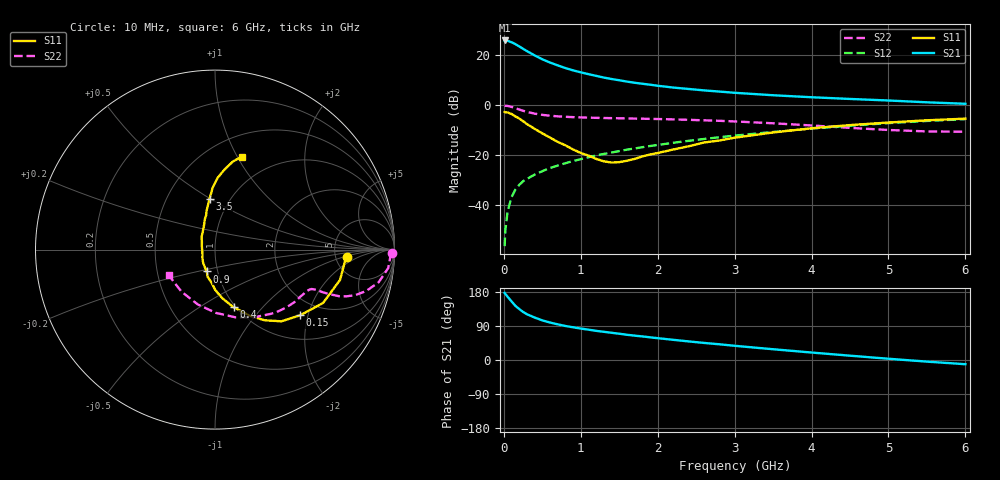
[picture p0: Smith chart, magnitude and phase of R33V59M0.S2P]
! SIEMENS Small Signal Semiconductors
! BFR181
! Si NPN RF Bipolar Junction Transistor in SOT23
! VCE = 3.5 V  IC = 9 mA
! Common Emitter S-Parameters:  May  1996
# GHz  S  MA  R  50
!  f  S11  S21  S12  S22
! GHz  MAG  ANG  MAG  ANG  MAG  ANG  MAG  ANG
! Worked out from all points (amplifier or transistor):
!   36 points, 10 MHz to 6 GHz, reference 50 ohm
!   highest |S21| = 26.0 dB at 10 MHz (marker M1)
!   |S21| within 3 dB of that: start of sweep to 232.2 MHz
!   unconditionally stable (mu >= 1): 819.5 MHz to 2.688 GHz
!   at 250 MHz: K = 0.58, MSG = 26.5 dB, |S12| = -30.4 dB
!   at 1.4 GHz: K = 1.06, MAG = 13.2 dB, |S12| = -18.9 dB
!   at 6 GHz: K = 0.85, MSG = 3.1 dB, |S12| = -5.5 dB
!   S11 on the Smith chart (normalised r, x): 10 MHz: 6.36, -1.06; 150 MHz: 1.56, -1.79; 400 MHz: 0.98, -0.71; 900 MHz: 0.89, -0.22; 3.5 GHz: 0.80, +0.50; 6 GHz: 0.72, +1.05
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0.01  0.735 -3.0  19.95 177.0  0.0015 82.7  0.9858 -1.1
0.02  0.7261 -5.6  19.92 174.2  0.0032 91.7  0.9774 -2.5
0.05  0.717 -13.6  19.6 166.6  0.0076 84.2  0.9705 -6.1
0.1  0.6715 -26.3  18.35 154.6  0.0144 77.2  0.9297 -11.3
0.15  0.5994 -37.6  16.83 142.9  0.0204 73.1  0.8737 -15.3
0.2  0.5446 -47.2  15.16 134.5  0.0254 71.1  0.8231 -17.9
0.25  0.4806 -55.0  13.59 126.9  0.0301 68.6  0.777 -19.6
0.3  0.421 -61.7  12.21 120.8  0.0334 67.9  0.7379 -20.6
0.4  0.3376 -72.1  10.03 112.1  0.0408 67.3  0.6807 -21.3
0.5  0.2742 -81.4  8.355 104.5  0.0478 67.7  0.6437 -21.6
0.6  0.2254 -89.6  7.209 98.9  0.0553 68.1  0.6185 -21.6
0.7  0.1848 -96.0  6.316 94.1  0.0619 68.9  0.601 -21.8
0.8  0.1577 -105.0  5.585 89.8  0.069 68.8  0.5883 -22.0
0.9  0.1302 -110.8  5.021 86.3  0.0763 69.2  0.5791 -22.3
1.1  0.0981 -132.7  4.214 80.1  0.0909 69.3  0.5658 -23.7
1.3  0.0753 -157.8  3.597 74.4  0.106 69.1  0.5563 -25.3
1.6  0.0773 161.9  2.988 66.6  0.1291 68.3  0.5453 -28.2
2.2  0.1297 120.5  2.272 53.3  0.1771 65.3  0.5217 -35.9
3.5  0.2853 96.1  1.591 28.4  0.2924 54.9  0.4364 -59.7
4.5  0.4012 87.8  1.341 11.4  0.3903 44.0  0.3527 -89.2
5.5  0.5009 78.5  1.148 -4.3  0.4854 31.2  0.2995 -128.8
6  0.5401 73.8  1.073 -11.1  0.5281 24.0  0.2948 -150.7
